|   IBIS Model for C5517
[IBIS ver]   4.1
[File name]   sprm632.ibs
[File Rev]   1.0
[Notes]
   IBIS model regenerated with the latest tool
[Date]   Mar 26, 2012
[Source]   TI
[Disclaimer] Please be aware that in the absence of a written agreement,
   Texas Instruments (TI) assumes no liability for: 1) the
   accuracy of the IBIS models provided to your company, 2) the
   proper functioning of these IBIS models in your design or for
   any resulting applications, or; 3) infringement of patents,
   copyrights, or intellectual property rights resulting from
   your use of these IBIS models. TI provides IBIS models as a
   service to our customers and therefore reserves the right to
   limit distribution of the IBIS models.
[Copyright]   Property of Texas Instruments Incorporated. Unauthorized
   reproduction and/or distribution is strictly prohibited. This
   product is protected under copyright law and trade secret law
   as an unpublished work. Copyright (C) 2011, Texas Instruments
   Incorporated, all rights reserved. These commodities are under
   the U.S. Government distribution license control. As such,
   they are not to be re-exported without the prior approval of
   the U.S. Department of Commerce.
|[Notes]
| - Signal names correspond to names in C5515 Data Manual Section 3.4.   |
| - Some IV curves contain Non monotonic data points.   |
|   File passes ibischk5 version 5.0.3
|   IBIS Quality Notes
|IBISCHK5 V5.0.3
|Checking Y:\corazon_phoenix_ibis\c5517.ibs for IBIS 4.2 Compatibility...
|WARNING - Model Model_1: POWER Clamp : Maximum value never becomes zero
|WARNING - Model Model_5: POWER Clamp : Maximum value never becomes zero
|WARNING - Model Model_7: POWER Clamp : Maximum value never becomes zero
|WARNING - Model Model_9: POWER Clamp : Maximum value never becomes zero
|WARNING - Model Model_11: POWER Clamp : Maximum value never becomes zero
|WARNING - Model Model_15: POWER Clamp : Maximum value never becomes zero
|WARNING - Model Model_25: POWER Clamp : Maximum value never becomes zero
|WARNING - Model Model_29: POWER Clamp : Maximum value never becomes zero
|WARNING - Model Model_31: POWER Clamp : Maximum value never becomes zero
|WARNING - Model Model_33: POWER Clamp : Maximum value never becomes zero
|WARNING - Model Model_35: POWER Clamp : Maximum value never becomes zero
|WARNING - Model Model_39: POWER Clamp : Maximum value never becomes zero
|WARNING - Model Model_41: GND Clamp : Maximum value never becomes zero
|WARNING - Model Model_45: GND Clamp : Maximum value never becomes zero
|WARNING - Model Model_47: GND Clamp : Maximum value never becomes zero
|WARNING - Model Model_49: GND Clamp : Maximum value never becomes zero
|WARNING - Model Model_51: GND Clamp : Maximum value never becomes zero
|WARNING - Model Model_55: GND Clamp : Maximum value never becomes zero
|WARNING - Model Model_65: POWER Clamp : Maximum value never becomes zero
|WARNING - Model Model_67: POWER Clamp : Maximum value never becomes zero
|WARNING - Model Model_73: POWER Clamp : Maximum value never becomes zero
|WARNING - Model Model_75: POWER Clamp : Maximum value never becomes zero
|WARNING - Model Model_77: POWER Clamp : Maximum value never becomes zero
|WARNING - Model Model_79: POWER Clamp : Maximum value never becomes zero
|WARNING - Model Model_81: POWER Clamp : Maximum value never becomes zero
|WARNING - Model Model_83: POWER Clamp : Maximum value never becomes zero
|WARNING - Model Model_85: POWER Clamp : Maximum value never becomes zero
|WARNING - Model Model_87: POWER Clamp : Maximum value never becomes zero
|WARNING - Model Model_93: POWER Clamp : Maximum value never becomes zero
|WARNING - Model Model_95: POWER Clamp : Maximum value never becomes zero
|WARNING - Model Model_105: GND Clamp : Maximum value never becomes zero
|WARNING - Model Model_109: GND Clamp : Maximum value never becomes zero
|WARNING - Model Model_111: GND Clamp : Maximum value never becomes zero
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[Component]   C5517
[Manufacturer]   Texas Instruments
| Source IO level model revisions
|Model   Revision   Date
|OC3350CT   1.0   Dec 28, 2011
|IC33THYPD   1.0   Dec 22, 2011
|BC3350CTHYPU   1.0   Dec 27, 2011
|BC3350CTHYPD   1.0   Dec 27, 2011
|BI2C33S   1.0   Dec 28, 2011
|BI2C33T   1.0   Dec 23, 2011
|BC3340CTSCHYPD   1.0   Dec 27, 2011
|IC33THYPU   1.0   Dec 22, 2011
[Package]
|   typ   min   max
R_pkg   0.1827   8.34E-02   2.82E-01
L_pkg   2.685E-09   1.26E-09   4.11E-09
C_pkg   1.0325E-12   5.05E-13   1.56E-12
[Pin]   signal_name   model_name   R_pin   L_pin   C_pin
F14   #N   NC
A12   ANA_LDOO   NC
B13   BG_CAP   NC
C7   CLK_SEL   Selector_3   2.03E-01   2.65E-09   1.22E-12
A8   CLKIN   Selector_3   1.85E-01   3.14E-09   7.97E-13
A7   CLKOUT   Selector_4   2.10E-01   3.01E-09   6.50E-13
D12   DSP_LDO_EN   NC
E10   DSP_LDOO   NC
C4   EM_D11   Selector_6   2.39E-01   2.98E-09   8.05E-13
L1   EM_A13   Selector_6   2.07E-01   3.17E-09   7.07E-13
C1   EM_A4   Selector_6   1.67E-01   3.20E-09   7.67E-13
K6   EM_WAIT3   Selector_6   2.33E-01   3.46E-09   1.30E-12
N1   EM_A15_GP21   Selector_6   2.39E-01   3.42E-09   5.97E-13
K1   EM_A12_CLE   Selector_6   2.00E-01   3.12E-09   6.76E-13
E1   EM_A2   Selector_6   1.91E-01   2.92E-09   7.13E-13
C3   EM_CS4   Selector_6   2.23E-01   2.73E-09   7.77E-13
K4   EM_D13   Selector_6   1.10E-01   1.50E-09   7.10E-13
E5   EM_D1   Selector_6   1.32E-01   2.27E-09   1.25E-12
B3   EM_CS0   Selector_6   2.18E-01   2.72E-09   6.77E-13
H3   EM_D7   Selector_6   9.97E-02   1.51E-09   6.15E-13
E2   EM_A16_GP22   Selector_6   1.28E-01   2.26E-09   8.17E-13
C5   EM_CS2   Selector_6   1.40E-01   1.77E-09   8.20E-13
J4   EM_D15   Selector_6   2.11E-01   3.00E-09   8.75E-13
B1   EM_BA1   Selector_6   1.69E-01   3.26E-09   8.03E-13
G2   EM_A18_GP24   Selector_6   2.10E-01   3.09E-09   6.98E-13
B2   EM_A0   Selector_6   2.10E-01   2.89E-09   5.81E-13
E3   EM_D8   Selector_6   2.36E-01   3.60E-09   8.20E-13
D1   EM_A5   Selector_6   2.00E-01   3.07E-09   7.12E-13
M2   EM_D5   Selector_6   1.24E-01   2.10E-09   1.01E-12
H2   EM_A7   Selector_6   2.13E-01   3.13E-09   6.67E-13
J2   EM_A9   Selector_6   1.65E-01   2.08E-09   8.02E-13
N2   EM_SDCKE   Selector_6   1.74E-01   3.20E-09   9.99E-13
G4   EM_A19_GP25   Selector_6   2.06E-01   2.82E-09   7.99E-13
G1   EM_WAIT4   Selector_6   1.46E-01   2.80E-09   7.40E-13
K5   EM_D6   Selector_6   1.30E-01   2.01E-09   1.13E-12
H1   EM_WE   Selector_6   1.46E-01   2.87E-09   6.78E-13
C2   EM_A1   Selector_6   1.85E-01   2.63E-09   6.84E-13
M3   EM_SDCLK   Selector_6   2.02E-01   2.70E-09   8.45E-13
F1   EM_A6   Selector_6   1.86E-01   2.87E-09   6.26E-13
D4   EM_D3   Selector_6   1.76E-01   2.40E-09   1.01E-12
D2   EM_A3   Selector_6   1.33E-01   2.35E-09   7.63E-13
A6   EM_SDRAS   Selector_6   2.11E-01   2.91E-09   6.68E-13
H4   EM_WAIT5   Selector_6   1.84E-01   2.36E-09   9.32E-13
L2   EM_A10   Selector_6   1.18E-01   1.93E-09   8.47E-13
J1   EM_A8   Selector_6   1.47E-01   2.82E-09   7.20E-13
D5   EM_WAIT2   Selector_6   2.73E-01   3.58E-09   1.15E-12
A1   EM_BA0   Selector_6   2.33E-01   3.78E-09   6.59E-13
F4   EM_D9   Selector_6   1.29E-01   1.81E-09   9.00E-13
J3   EM_A20_GP26   Selector_6   1.62E-01   2.58E-09   1.25E-12
D3   EM_D10   Selector_6   2.47E-01   3.77E-09   9.20E-13
L3   EM_D12   Selector_6   2.03E-01   2.77E-09   7.35E-13
M4   EM_CS3   Selector_6   1.33E-01   1.97E-09   8.96E-13
F3   EM_D2   Selector_6   1.68E-01   2.02E-09   8.37E-13
E4   EM_OE   Selector_6   1.15E-01   1.51E-09   9.68E-13
P1   EM_DQM1   Selector_6   2.02E-01   3.74E-09   9.11E-13
B4   EM_SDCAS   Selector_6   2.79E-01   4.04E-09   8.65E-13
G3   EM_D0   Selector_6   1.52E-01   2.15E-09   1.06E-12
K3   EM_D14   Selector_6   1.95E-01   2.55E-09   7.29E-13
L4   EM_D4   Selector_6   1.18E-01   1.70E-09   9.84E-13
K2   EM_A11_ALE   Selector_6   1.34E-01   2.33E-09   7.16E-13
B6   EM_RNW   Selector_6   1.41E-01   2.06E-09   7.85E-13
F2   EM_A17_GP23   Selector_6   1.04E-01   1.77E-09   7.80E-13
A3   EM_CS5   Selector_6   2.10E-01   3.78E-09   8.09E-13
M1   EM_A14   Selector_6   2.06E-01   2.89E-09   5.82E-13
A4   EM_CS1   Selector_6   1.74E-01   2.97E-09   7.26E-13
B5   EM_DQM0   Selector_6   2.45E-01   3.21E-09   7.61E-13
L6   EMU0   Selector_2   9.20E-02   1.26E-09   9.54E-13
M5   EMU1   Selector_2   1.59E-01   2.01E-09   7.80E-13
D10   GPAIN0   NC
A11   GPAIN1   NC
B11   GPAIN2   NC
C11   GPAIN3   NC
C6   INT0N   Selector_7   2.40E-01   3.00E-09   1.13E-12
E7   INT1N   Selector_7   2.82E-01   4.11E-09   1.56E-12
P9   LCD_D5_GP15   Selector_4   1.66E-01   2.73E-09   5.96E-13
P12   LCD_D11_I2S2_DX_GP27_SPI_TX Selector_4   1.63E-01   2.44E-09   5.05E-13
N13   LCD_D14_UART_RXD_GP30_I2S3_RX Selector_4   1.40E-01   2.70E-09   7.84E-13
P14   LCD_D15_UART_TXD_GP31_I2S3_DX Selector_4   1.51E-01   3.07E-09   6.72E-13
P11   LCD_D9_I2S2_FS_GP19_SPI_CS0 Selector_4   1.36E-01   2.87E-09   7.14E-13
P6   LCD_D0_SPI_RX   Selector_4   1.68E-01   2.77E-09   6.88E-13
P5   LCD_RW_WRB_SPI_CS2   Selector_4   1.77E-01   2.90E-09   7.33E-13
N5   LCD_RS_SPI_CS3   Selector_4   1.14E-01   2.01E-09   7.53E-13
N3   LCD_EN_RDB_SPI_CLK   Selector_4   1.66E-01   3.02E-09   8.89E-13
N9   LCD_D6_GP16   Selector_4   1.26E-01   2.21E-09   7.81E-13
N4   LCD_CS1_E1_SPI_CS1   Selector_4   1.61E-01   2.21E-09   5.99E-13
N10   LCD_D8_I2S2_CLK_GP18_SPI_CLK Selector_4   1.15E-01   2.40E-09   8.58E-13
P4   LCD_CS0_E0_SPI_CS0   Selector_4   1.40E-01   2.87E-09   7.71E-13
N12   LCD_D12_UART_RTS_GP28_I2S3_CLK Selector_4   1.77E-01   3.41E-09   7.41E-13
N7   LCD_D3_GP13   Selector_4   1.40E-01   1.97E-09   6.29E-13
N8   LCD_D4_GP14   Selector_4   1.41E-01   2.04E-09   7.00E-13
P7   LCD_D2_GP12   Selector_4   1.24E-01   2.50E-09   7.10E-13
P10   LCD_D7_GP17   Selector_4   1.31E-01   2.64E-09   8.11E-13
P13   LCD_D13_UART_CTS_GP29_I2S3_FS Selector_4   2.10E-01   3.20E-09   5.66E-13
N11   LCD_D10_I2S2_RX_GP20_SPI_RX Selector_4   1.52E-01   2.25E-09   6.62E-13
N6   LCD_D1_SPI_TX   Selector_4   1.10E-01   2.01E-09   7.72E-13
B12   LDOI   NC
F13   LDOI   NC
D6   RESETN   Selector_7   1.73E-01   2.47E-09   1.33E-12
C12   RSV0   NC
J10   RSV1   NC
J11   RSV1   NC
D14   RSV3   NC
C14   RSV4   NC
C13   RSV5   NC
D8   RTC_CLKOUT   Selector_1   1.82E-01   2.62E-09   1.34E-12
B9   RTC_XI   NC
A9   RTC_XO   NC
B7   SCL   Selector_5   8.34E-02   1.45E-09   6.42E-13
M10   SD0_D1_I2S0_RX_GP3   Selector_4   2.12E-01   3.53E-09   8.62E-13
L10   SD0_CLK_I2S0_CKL_GP0 Selector_4   1.21E-01   2.10E-09   1.26E-12
M11   SD0_CMD_I2S0_FS_GP1  Selector_4   1.09E-01   1.70E-09   7.27E-13
L11   SD0_D3_GP5   Selector_4   1.94E-01   2.78E-09   1.14E-12
L9   SD0_D0_I2S0_DX_GP2   Selector_4   1.32E-01   2.04E-09   1.24E-12
L12   SD0_D2_GP4   Selector_4   2.45E-01   3.56E-09   7.75E-13
L13   SD1_D3_GP11   Selector_4   1.36E-01   2.30E-09   6.70E-13
M13   SD1_CLK_I2S1_CLK_GP6 Selector_4   1.83E-01   2.54E-09   5.51E-13
M12   SD1_D1_I2S1_RX_GP9   Selector_4   2.23E-01   3.66E-09   7.57E-13
M14   SD1_D0_I2S1_DX_GP8   Selector_4   1.64E-01   3.07E-09   5.83E-13
K14   SD1_D2_GP10   Selector_4   1.58E-01   3.08E-09   6.45E-13
L14   SD1_CMD_I2S1_FS_GP7  Selector_4   1.90E-01   3.10E-09   5.39E-13
B8   SDA   Selector_5   2.37E-01   3.53E-09   7.21E-13
M6   TCK   Selector_7   1.49E-01   1.90E-09   8.84E-13
L7   TDI   Selector_7   1.09E-01   1.70E-09   1.08E-12
M7   TDO   Selector_2   1.69E-01   2.20E-09   9.82E-13
L8   TMS   Selector_7   1.66E-01   2.15E-09   9.72E-13
M9   TRSTN   Selector_3   1.44E-01   1.93E-09   8.03E-13
G9   USB_R1   NC
H9   USB_VSSA1P3   NC
J13   USB_VDD1P3   NC
H13   USB_VSS1P3   NC
G8   USB_VDDPLL   NC
F11   USB_VSSOSC   NC
G11   USB_VSSPLL   NC
J12   USB_VBUS   NC
F12   USB_LDOO   NC
G10   USB_VSSREF   NC
H12   USB_VDDA3P3   NC
J14   USB_DM   NC
H14   USB_DP   NC
H10   USB_VDDA1P3   NC
G12   USB_VDDOSC   NC
G14   USB_MXO   NC
H11   USB_VSS3P3   NC
G13   USB_MXI   NC
A10   VDDA_ANA   NC
C10   VDDA_PLL   NC
F6   VDDC   NC
H8   VDDC   NC
J6   VDDC   NC
K10   VDDC   NC
L5   VDDC   NC
F7   VDDIO1   NC
K12   VDDIO1   NC
K7   VDDIO1   NC
N14   VDDIO1   NC
P3   VDDIO1   NC
P8   VDDIO1   NC
A2   VDDIO2   NC
A5   VDDIO2   NC
E6   VDDIO2   NC
F5   VDDIO2   NC
G5   VDDIO2   NC
H5   VDDIO2   NC
H7   VDDIO2   NC
J5   VDDIO2   NC
P2   VDDIO2   NC
F8   VDDIO4   NC
C8   VDDRTC   NC
A13   VSS   NC
A14   VSS   NC
D11   VSS   NC
D13   VSS   NC
D7   VSS   NC
E11   VSS   NC
E12   VSS   NC
E13   VSS   NC
E14   VSS   NC
E9   VSS   NC
F10   VSS   NC
F9   VSS   NC
G6   VSS   NC
G7   VSS   NC
H6   VSS   NC
J7   VSS   NC
J8   VSS   NC
J9   VSS   NC
K11   VSS   NC
K13   VSS   NC
K8   VSS   NC
K9   VSS   NC
B10   VSSA_ANA   NC
B14   VSSA_ANA   NC
D9   VSSA_PLL   NC
C9   VSSRTC   NC
E8   WAKEUP   Selector_8   2.07E-01   3.19E-09   1.42E-12
M8   XF   Selector_2   8.38E-02   1.35E-09   8.20E-13
|   Usage OUTPUT#1.8V/2.75V/3.3V###OC3350CT.PAD
|   Base model OC3350CT
[Model Selector] Selector_1
Model_17 3-STATE,2.75V
Model_19 3-STATE,1.8V
Model_20 3-STATE,3.3V
Model_21 3-STATE,2.75V
Model_22 3-STATE,1.8V
Model_24 3-STATE,3.3V
|   Usage I/O#1.8V/2.75V/3.3V#PU/PU_OFF##BC3350CTHYPU.PAD
|   Base model BC3350CTHYPU
[Model Selector] Selector_2
Model_41 I/O,2.75V,PU,IND
Model_42 I/O,2.75V,PU_OFF,IND
Model_45 I/O,1.8V,PU,COM
Model_46 I/O,1.8V,PU_OFF,COM
Model_47 I/O,3.3V,PU,COM
Model_48 I/O,3.3V,PU_OFF,COM
Model_49 I/O,2.75V,PU,COM
Model_50 I/O,2.75V,PU_OFF,COM
Model_51 I/O,1.8V,PU,IND
Model_52 I/O,1.8V,PU_OFF,IND
Model_55 I/O,3.3V,PU,IND
Model_56 I/O,3.3V,PU_OFF,IND
|   Usage INPUT#1.8V/2.75V/3.3V#PD/PD_OFF##IC33THYPD.PAD
|   Base model IC33THYPD
[Model Selector] Selector_3
Model_1 INPUT,2.75V,PD,IND
Model_10 INPUT,2.75V,PD_OFF,COM
Model_11 INPUT,1.8V,PD,IND
Model_12 INPUT,1.8V,PD_OFF,IND
Model_15 INPUT,3.3V,PD,IND
Model_16 INPUT,3.3V,PD_OFF,IND
Model_2 INPUT,2.75V,PD_OFF,IND
Model_5 INPUT,1.8V,PD,COM
Model_6 INPUT,1.8V,PD_OFF,COM
Model_7 INPUT,3.3V,PD,COM
Model_8 INPUT,3.3V,PD_OFF,COM
Model_9 INPUT,2.75V,PD,COM
|   Usage I/O#1.8V/2.75V/3.3V#PD/PD_OFF##BC3350CTHYPD.PAD
|   Base model BC3350CTHYPD
[Model Selector] Selector_4
Model_25 I/O,2.75V,PD,IND
Model_26 I/O,2.75V,PD_OFF,IND
Model_29 I/O,1.8V,PD,COM
Model_30 I/O,1.8V,PD_OFF,COM
Model_31 I/O,3.3V,PD,COM
Model_32 I/O,3.3V,PD_OFF,COM
Model_33 I/O,2.75V,PD,COM
Model_34 I/O,2.75V,PD_OFF,COM
Model_35 I/O,1.8V,PD,IND
Model_36 I/O,1.8V,PD_OFF,IND
Model_39 I/O,3.3V,PD,IND
Model_40 I/O,3.3V,PD_OFF,IND
|   Usage I/O#1.8V/2.75V/3.3V###BI2C33T.PAD
|   Base model BI2C33T
[Model Selector] Selector_5
Model_100 I/O_OPEN_DRAIN,3.3V
Model_101 I/O_OPEN_DRAIN,2.75V
Model_102 I/O_OPEN_DRAIN,1.8V
Model_104 I/O_OPEN_DRAIN,3.3V
Model_97 I/O_OPEN_DRAIN,2.75V
Model_99 I/O_OPEN_DRAIN,1.8V
|   Usage I/O#1.8V/2.75V/3.3V#PD/PD_OFF##BC3340CTSCHYPD.PAD
|   Base model BC3340CTSCHYPD
[Model Selector] Selector_6
Model_65 I/O,2.75V,PD,IND
Model_66 I/O,2.75V,PD_OFF,IND
Model_67 I/O,2.75V,PD,IND
Model_68 I/O,2.75V,PD_OFF,IND
Model_73 I/O,1.8V,PD,COM
Model_74 I/O,1.8V,PD_OFF,COM
Model_75 I/O,1.8V,PD,COM
Model_76 I/O,1.8V,PD_OFF,COM
Model_77 I/O,3.3V,PD,COM
Model_78 I/O,3.3V,PD_OFF,COM
Model_79 I/O,3.3V,PD,COM
Model_80 I/O,3.3V,PD_OFF,COM
Model_81 I/O,2.75V,PD,COM
Model_82 I/O,2.75V,PD_OFF,COM
Model_83 I/O,2.75V,PD,COM
Model_84 I/O,2.75V,PD_OFF,COM
Model_85 I/O,1.8V,PD,IND
Model_86 I/O,1.8V,PD_OFF,IND
Model_87 I/O,1.8V,PD,IND
Model_88 I/O,1.8V,PD_OFF,IND
Model_93 I/O,3.3V,PD,IND
Model_94 I/O,3.3V,PD_OFF,IND
Model_95 I/O,3.3V,PD,IND
Model_96 I/O,3.3V,PD_OFF,IND
|   Usage INPUT#1.8V/2.75V/3.3V#PU/PU_OFF##IC33THYPU.PAD
|   Base model IC33THYPU
[Model Selector] Selector_7
Model_105 INPUT,2.75V,PU,IND
Model_106 INPUT,2.75V,PU_OFF,IND
Model_109 INPUT,1.8V,PU,COM
Model_110 INPUT,1.8V,PU_OFF,COM
Model_111 INPUT,3.3V,PU,COM
Model_112 INPUT,3.3V,PU_OFF,COM
Model_113 INPUT,2.75V,PU,COM
Model_114 INPUT,2.75V,PU_OFF,COM
Model_115 INPUT,1.8V,PU,IND
Model_116 INPUT,1.8V,PU_OFF,IND
Model_119 INPUT,3.3V,PU,IND
Model_120 INPUT,3.3V,PU_OFF,IND
|   Usage I/O#1.8V/2.75V/3.3V###BI2C33S.PAD
|   Base model BI2C33S
[Model Selector] Selector_8
Model_57 I/O_OPEN_DRAIN,2.75V
Model_59 I/O_OPEN_DRAIN,1.8V
Model_60 I/O_OPEN_DRAIN,3.3V
Model_61 I/O_OPEN_DRAIN,2.75V
Model_62 I/O_OPEN_DRAIN,1.8V
Model_64 I/O_OPEN_DRAIN,3.3V
| Models and submodels in the file (90): Model_1 (Input), Model_2 (Input), Model_5 (Input), Model_6 (Input), Model_7 (Input), Model_8 (Input), Model_9 (Input), Model_10 (Input), Model_11 (Input), Model_12 (Input), Model_15 (Input), Model_16 (Input), Model_17 (3-state), Model_19 (3-state), Model_20 (3-state), Model_21 (3-state), Model_22 (3-state), Model_24 (3-state), Model_25 (I/O), Model_26 (I/O), Model_29 (I/O), Model_30 (I/O), Model_31 (I/O), Model_32 (I/O), Model_33 (I/O), Model_34 (I/O), Model_35 (I/O), Model_36 (I/O), Model_39 (I/O), Model_40 (I/O), Model_41 (I/O), Model_42 (I/O), Model_45 (I/O), Model_46 (I/O), Model_47 (I/O), Model_48 (I/O), Model_49 (I/O), Model_50 (I/O), Model_51 (I/O), Model_52 (I/O), Model_55 (I/O), Model_56 (I/O), Model_57 (I/O_open_drain), Model_59 (I/O_open_drain), Model_60 (I/O_open_drain), Model_61 (I/O_open_drain), Model_62 (I/O_open_drain), Model_64 (I/O_open_drain), Model_65 (I/O), Model_66 (I/O), Model_67 (I/O), Model_68 (I/O), Model_73 (I/O), Model_74 (I/O), Model_75 (I/O), Model_76 (I/O), Model_77 (I/O), Model_78 (I/O), Model_79 (I/O), Model_80 (I/O), Model_81 (I/O), Model_82 (I/O), Model_83 (I/O), Model_84 (I/O), Model_85 (I/O), Model_86 (I/O), Model_87 (I/O), Model_88 (I/O), Model_93 (I/O), Model_94 (I/O), Model_95 (I/O), Model_96 (I/O), Model_97 (I/O_open_drain), Model_99 (I/O_open_drain), Model_100 (I/O_open_drain), Model_101 (I/O_open_drain), Model_102 (I/O_open_drain), Model_104 (I/O_open_drain), Model_105 (Input), Model_106 (Input)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
